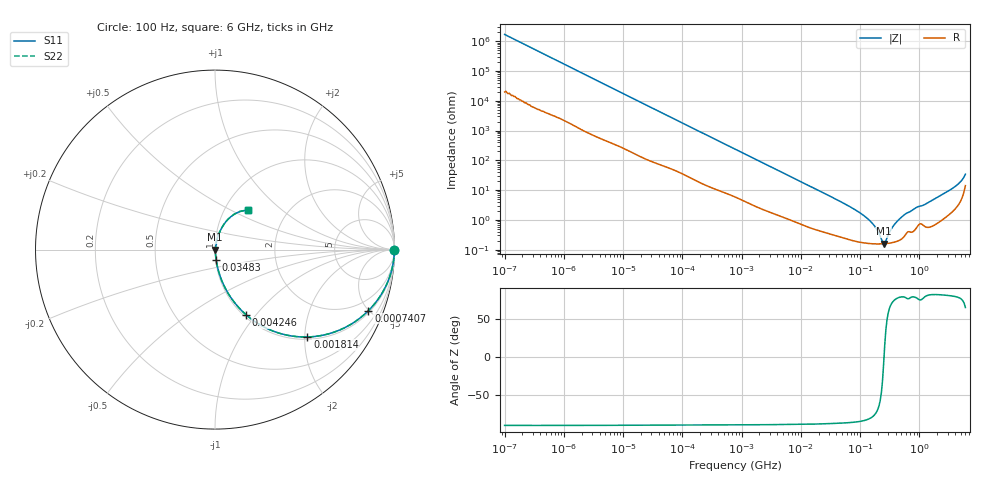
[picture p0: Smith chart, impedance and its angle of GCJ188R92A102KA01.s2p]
!Murata Part Number: GCJ188R92A102KA01
!These Parameters are Measured in Series Mode Connection
!Data Generated on Mar 13, 2026
!  o--ll--o
!Port1  Port2
!  o------o
!Operation Temp=25[degC], DC Bias Voltage=0[V]
!Freq. Start=100[Hz] Stop=6[GHz] 401[Steps]
# Hz S RI R 50
!Freq.(Hz) S11(Real) S11(Imag) S21(Real) S21(Imag) S12(Real) S12(Imag) S22(Real) S22(Imag)
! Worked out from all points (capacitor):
!   401 points, 100 Hz to 6 GHz, reference 50 ohm
!   read as one part in series: C = 938 pF near 109 Hz
!   lowest |Z| = 160 mohm at 249.8 MHz (marker M1)
!   series resonance near 253.8 MHz, so ESL is about 420 pH
!   S11 on the Smith chart (normalised r, x): 100 Hz: open; 740.7 kHz: 1.12, -4.97; 1.814 MHz: 1.05, -2.06; 4.246 MHz: 1.03, -0.89; 34.83 MHz: 1.01, -0.11; 6 GHz: 1.28, +0.62
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100  1 -5.92e-05  7e-07 5.92e-05  7e-07 5.92e-05  1 -5.92e-05
179  1 -0.000105  1.2e-06 0.000105  1.2e-06 0.000105  1 -0.000105
2008  1 -0.00116  1.56e-05 0.00116  1.56e-05 0.00116  1 -0.00116
40335  0.9991 -0.0227  0.000895 0.0227  0.000895 0.0227  0.9991 -0.0227
211427  0.9844 -0.1146  0.0156 0.1146  0.0156 0.1146  0.9844 -0.1146
740679  0.8548 -0.3402  0.1452 0.3402  0.1452 0.3402  0.8548 -0.3402
774597  0.8438 -0.3508  0.1562 0.3508  0.1562 0.3508  0.8438 -0.3508
1813585  0.5146 -0.4868  0.4854 0.4868  0.4854 0.4868  0.5146 -0.4868
4246196  0.1736 -0.3633  0.8264 0.3633  0.8264 0.3633  0.1736 -0.3633
1.555665e7  0.0201 -0.1213  0.9799 0.1213  0.9799 0.1213  0.0201 -0.1213
3.482834e7  0.0062 -0.0552  0.9938 0.0552  0.9938 0.0552  0.0062 -0.0552
8.154455e7  0.00242 -0.0221  0.9976 0.0221  0.9976 0.0221  0.00242 -0.0221
1.334425e8  0.00175 -0.011  0.9982 0.011  0.9982 0.011  0.00175 -0.011
1.825626e8  0.00159 -0.00537  0.9984 0.00537  0.9984 0.00537  0.00159 -0.00537
2.497637e8  0.00158 -0.000251  0.9984 0.000251  0.9984 0.000251  0.00158 -0.000251
2.731619e8  0.0016 0.00119  0.9984 -0.00119  0.9984 -0.00119  0.0016 0.00119
3.124326e8  0.00167 0.00339  0.9983 -0.00339  0.9983 -0.00339  0.00167 0.00339
3.908258e8  0.00187 0.00724  0.9981 -0.00724  0.9981 -0.00724  0.00187 0.00724
5.59173e8  0.00301 0.0145  0.997 -0.0145  0.997 -0.0145  0.00301 0.0145
3.352442e9  0.026 0.0979  0.974 -0.0979  0.974 -0.0979  0.026 0.0979
4.796499e9  0.0624 0.1575  0.9376 -0.1575  0.9376 -0.1575  0.0624 0.1575
6e9  0.1848 0.2218  0.8152 -0.2218  0.8152 -0.2218  0.1848 0.2218
